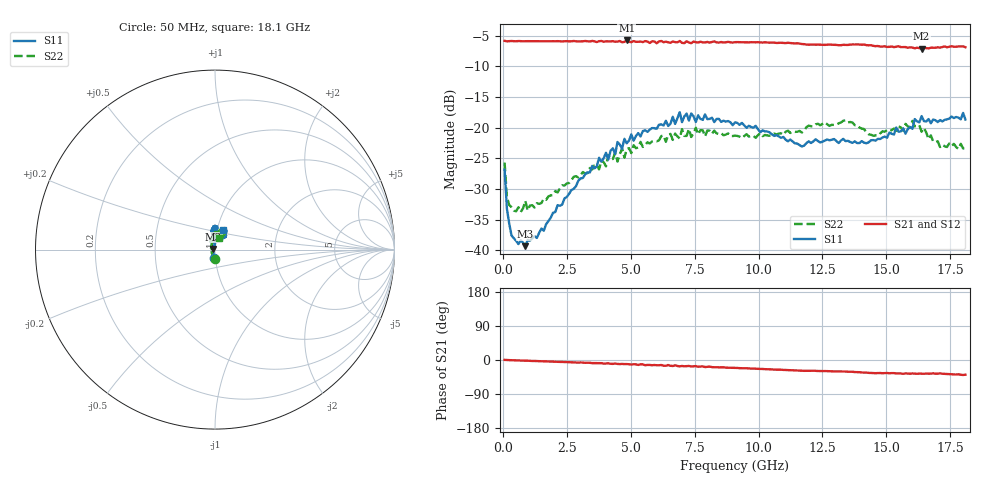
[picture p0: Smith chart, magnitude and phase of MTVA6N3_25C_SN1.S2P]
! Network Analyzer HP8720D.06.14 Serial No. US36140669
!  5 Jul 2005  09:41:02
! Frequency  S11  S21  S12  S22
# HZ  S  DB R 50
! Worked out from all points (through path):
!   201 points, 50 MHz to 18.1 GHz, reference 50 ohm
!   highest |S21| = -5.78 dB at 4.833 GHz (marker M1); lowest = -7.1 dB at 16.39 GHz (marker M2)
!   group delay of S21, straight-line fit = 6.23 ps
!   lowest |S11| = -39.3 dB at 862.2 MHz (marker M3), VSWR 1.02, Z = 49 + j0.397 ohm
!   |S11| at or under -10 dB: start of sweep to end of sweep
!   |S22| runs from -33.7 to -18.8 dB; largest |S21 - S12| = 0.017
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5e7  -26.83 -95.9  -5.84 0.3  -5.86 0.4  -25.67 -87.7
1.4025e8  -33.22 -112.6  -5.92 -0.1  -5.90 -0.0  -31.26 -129.7
3.2075e8  -37.56 -141.9  -5.86 -0.5  -5.89 -0.4  -32.95 -156.9
6.8175e8  -38.32 176.1  -5.89 -1.4  -5.91 -1.4  -33.72 179.4
8.6225e8  -39.30 158.1  -5.89 -1.8  -5.91 -1.7  -31.90 173.8
1.22325e9  -37.68 142.7  -5.91 -2.6  -5.92 -2.7  -33.01 156.6
3.1185e9  -28.18 92.7  -5.91 -6.8  -5.93 -7.1  -27.22 123.5
4.382e9  -24.31 84.7  -5.98 -9.2  -5.93 -10.2  -24.04 111.8
4.47225e9  -22.32 80.9  -5.96 -10.3  -5.91 -9.6  -25.52 113.6
4.83325e9  -22.53 89.8  -5.78 -10.7  -5.88 -11.5  -23.49 100.1
6.09675e9  -19.51 85.1  -5.93 -13.9  -5.88 -13.9  -22.06 95.8
6.7285e9  -19.38 91.2  -6.05 -14.0  -6.19 -14.9  -20.95 90.1
6.909e9  -17.46 90.1  -5.86 -16.8  -6.00 -15.9  -21.74 87.5
6.99925e9  -19.09 89.4  -6.16 -15.7  -6.20 -17.0  -20.23 89.5
7.36025e9  -17.67 84.3  -6.22 -17.1  -6.06 -16.3  -21.51 94.1
7.54075e9  -19.07 86.5  -6.06 -16.1  -5.93 -17.9  -20.00 93.1
9.075e9  -19.12 98.3  -6.06 -20.8  -6.04 -20.9  -21.29 81.4
1.21435e10  -22.22 89.0  -6.44 -28.3  -6.41 -28.6  -19.76 77.4
1.512175e10  -20.78 52.5  -6.82 -35.0  -6.70 -34.8  -20.55 77.6
1.602425e10  -20.17 60.4  -6.93 -35.5  -7.05 -37.1  -18.87 66.6
1.638525e10  -18.10 58.4  -7.13 -36.2  -6.96 -35.9  -20.65 59.9
1.81e10  -18.65 67.3  -6.88 -38.8  -6.96 -39.8  -23.39 72.6
